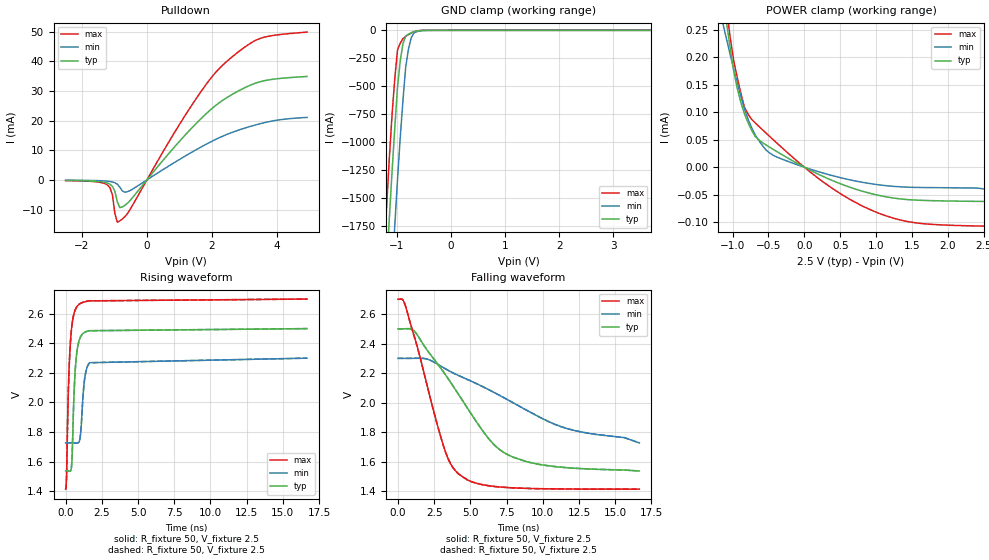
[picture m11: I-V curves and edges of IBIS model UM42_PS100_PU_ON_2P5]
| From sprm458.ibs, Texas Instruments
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|IDG09_OUM42_PS100_PU_OFF_2P75; BUFFER IN NORMAL MODE WITH PULLUP OFF
|   Model Cell UM42_PS100_PU_ON_2P5
|IDG09_OUM42_PS100_PU_ON_2P5
[Model]   UM42_PS100_PU_ON_2P5
Model_type   I/O_open_drain
Polarity   Non-Inverting
Enable   Active-Low
Vinl =  0.7V
Vinh =  1.7V
Cref =  15pF
Rref =  100.00M
Vref =  0V
Vmeas =  1.25
C_comp   4.232p   4.190p   4.462p
[Model Spec]
Vinl   0.7V   0.7V   0.7V
Vinh   1.7V   1.7V   1.7V
[Temperature Range]   25   125   -40
[Voltage Range]   2.5   2.3   2.7
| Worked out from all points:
|   slope of the pulldown table from 0 to 0.375 V, typ, clamps not added: 74.6 ohm
|   GND clamp passes 1 mA (typ) near -0.53 V on its own axis
|   POWER clamp passes 1 mA (typ) near -1.78 V on its own axis
|   rising waveform, R_fixture 50, V_fixture 2.5: 20-80 % time 259ps typ, 279ps min, 259ps max; typ from 1.54 V to 2.5 V
|   rising waveform, R_fixture 50, V_fixture 2.5: 20-80 % time 259ps typ, 279ps min, 259ps max; typ from 1.54 V to 2.5 V
|   falling waveform, R_fixture 50, V_fixture 2.5: 20-80 % time 4.11ns typ, 6.99ns min, 2.12ns max; typ from 2.5 V to 1.54 V
|   falling waveform, R_fixture 50, V_fixture 2.5: 20-80 % time 4.11ns typ, 6.99ns min, 2.12ns max; typ from 2.5 V to 1.54 V
| Nom Voltages:
|   VDD=1.1, VDDS=2.5, VSS=0, VSSS=0
| Min Voltages:
|   VDD=1, VDDS=2.3, VSS=0, VSSS=0
| Max Voltages:
|   VDD=1.2, VDDS=2.7, VSS=0, VSSS=0
[POWER_clamp]
|   voltage   I(typ)   I(min)   I(max)
-2.5V     1.8mA      1.08mA     2.671mA
-1.136V   313.2uA    262.1uA    357.3uA
-1.086V   264.7uA    233.8uA    291.9uA
-1.035V   218.8uA    206.1uA    237.5uA
-934.3mV  143.7uA    152.9uA    162.6uA
-782.8mV  80.61uA    87uA       96.3uA
-580.8mV  44.38uA    38.8uA     67.78uA
-378.8mV  28.1uA     18.21uA    43.38uA
328.3mV   -20.7uA    -13.09uA   -32.87uA
984.8mV   -49.63uA   -31.07uA   -80.85uA
1.591V    -60uA      -36.78uA   -101.7uA
2.5V      -62.22uA   -39.5uA    -107.1uA
[Pulldown]
|   voltage   I(typ)   I(min)   I(max)
-2.5V     -180.8uA   -97.77uA   -227.7uA
-1.212V   -1.061mA   -434.4uA   -1.717mA
-1.061V   -2.159mA   -689.8uA   -4.966mA
-984.8mV  -3.82mA    -950.1uA   -11.34mA
-909.1mV  -7.402mA   -1.439mA   -14.27mA
-833.3mV  -9.346mA   -2.412mA   -13.85mA
-681.8mV  -8.607mA   -4.157mA   -12.46mA
-530.3mV  -7.118mA   -3.662mA   -10.23mA
1.212V    15.56mA    8.277mA    22.39mA
2.273V    26.42mA    14.48mA    38.13mA
3.409V    32.92mA    18.76mA    47.45mA
4.924V    34.93mA    21.1mA     49.91mA
[GND_clamp]
|   voltage   I(typ)   I(min)   I(max)
-2.5V     -14.76A    -15.63A    -14.26A
-1.237V   -2.586A    -3.523A    -2.036A
-1.187V   -2.133A    -3.066A    -1.587A
-1.136V   -1.687A    -2.615A    -1.149A
-1.035V   -874mA     -1.75A     -433mA
-984.8mV  -507.9mA   -1.335A    -176.7mA
-934.3mV  -271mA     -959.5mA   -114.6mA
-883.8mV  -118.6mA   -623.6mA   -73.68mA
-833.3mV  -50.91mA   -327.1mA   -53.8mA
-732.3mV  -22.27mA   -66.61mA   -24.29mA
-429.3mV  -157.7uA   -469.5uA   -130.6uA
5V        0A         0A         0A
[Ramp]
| variable   typ   min   max
dV/dt_f 0.57873053/4.1185315n 0.34403164/6.9944155n 0.77318457/2.1253239n
dV/dt_r 13.373859m/0.11353487n 10.179385m/0.18003826n 15.441486m/84.875314p
R_load = 50
[Rising Waveform]
R_fixture = 50
V_fixture = 2.5
V_fixture_min = 2.3
V_fixture_max = 2.7
|   time   V(typ)   V(min)   V(max)
0s        1.537V     1.727V     1.413V
66.89ps   1.537V     1.727V     1.503V
223ps     1.536V     1.727V     2.18V
354.2ps   1.538V     1.727V     2.436V
443.1ps   1.621V     1.727V     2.526V
657.9ps   2.208V     1.726V     2.625V
922.5ps   2.416V     1.733V     2.664V
1.307ns   2.474V     2.153V     2.681V
1.656ns   2.486V     2.269V     2.688V
16.67ns   2.5V       2.3V       2.7V
[Rising Waveform]
R_fixture = 50
V_fixture = 2.5
V_fixture_min = 2.3
V_fixture_max = 2.7
|   time   V(typ)   V(min)   V(max)
0s        1.537V     1.727V     1.413V
66.89ps   1.537V     1.727V     1.503V
223ps     1.536V     1.727V     2.18V
354.2ps   1.538V     1.727V     2.436V
443.1ps   1.621V     1.727V     2.526V
657.9ps   2.208V     1.726V     2.625V
922.5ps   2.416V     1.733V     2.664V
1.307ns   2.474V     2.153V     2.681V
1.656ns   2.486V     2.269V     2.688V
16.67ns   2.5V       2.3V       2.7V
[Falling Waveform]
R_fixture = 50
V_fixture = 2.5
V_fixture_min = 2.3
V_fixture_max = 2.7
|   time   V(typ)   V(min)   V(max)
0s        2.5V       2.3V       2.7V
320.4ps   2.5V       2.3V       2.698V
525.9ps   2.501V     2.3V       2.653V
1.206ns   2.476V     2.301V     2.423V
3.341ns   2.18V      2.225V     1.65V
4.221ns   2.05V      2.182V     1.514V
6.372ns   1.743V     2.083V     1.435V
7.937ns   1.631V     2V         1.422V
11.64ns   1.559V     1.825V     1.414V
16.67ns   1.537V     1.727V     1.413V
[Falling Waveform]
R_fixture = 50
V_fixture = 2.5
V_fixture_min = 2.3
V_fixture_max = 2.7
|   time   V(typ)   V(min)   V(max)
0s        2.5V       2.3V       2.7V
320.4ps   2.5V       2.3V       2.698V
525.9ps   2.501V     2.3V       2.653V
1.206ns   2.476V     2.301V     2.423V
3.341ns   2.18V      2.225V     1.65V
4.221ns   2.05V      2.182V     1.514V
6.372ns   1.743V     2.083V     1.435V
7.937ns   1.631V     2V         1.422V
11.64ns   1.559V     1.825V     1.414V
16.67ns   1.537V     1.727V     1.413V
